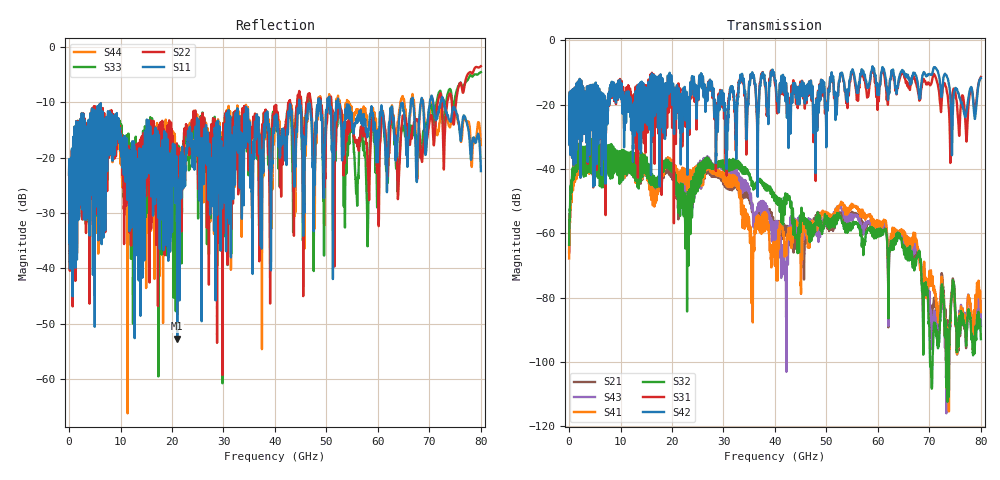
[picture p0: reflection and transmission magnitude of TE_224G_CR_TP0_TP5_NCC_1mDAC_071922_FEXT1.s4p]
!! Reference: tracy_3df_01a_2207
!! CHANNEL DESCRIPTION: TP0_TP5 CR Channel using 1meter DAC, CABLED NCC Host
!! MODEL DESCRIPTION: s4p, FEXT1
!! CONNECTOR DESCRIPTION: OSFP 200G OTB, NCC Socket
!! CABLE DESCRIPTION: 1meter 26AWG Cable
!! MODEL STATUS: Developmental
!! PORT DEFINITIONS:
!! Port  1  ----->  Side A  Side B  <-----  Port  2
!! Port  3  ----->  Side A  Side B  <-----  Port  4
# GHz S MA R 50
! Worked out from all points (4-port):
!   8000 points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, 10 MHz to 80 GHz, reference 50 ohm
!   strongest paths, dB at 10 MHz, 20.01 GHz, 40.01 GHz, 60.01 GHz, 80 GHz:
!     S42: -24.5, -18.5, -12.5, -15.2, -11.7
!     S31: -24.5, -26.1, -13.7, -17.6, -11.4
!     S32: -63.7, -39.3, -48.6, -60.8, -92.9
!     S41: -67.8, -38.5, -65.3, -58.1, -84.5
!     S43: -66.0, -38.7, -68.9, -59.4, -88.6
!     S21: -65.9, -41.3, -57.8, -59.5, -88.9
!   lowest |S11| = -52.7 dB at 21.01 GHz (marker M1), VSWR 1.00, Z = 50 + j0.231 ohm
!   |S11| at or under -10 dB: start of sweep to 44.68 GHz; 52.32 GHz to 66.38 GHz (14.06 GHz wide, 23.7 % of centre); 72.83 GHz to end of sweep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
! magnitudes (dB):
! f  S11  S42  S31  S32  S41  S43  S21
! 10 MHz  -23.1  -24.5  -24.5  -63.7  -67.8  -66.0  -65.9
! 1.96 GHz  -15.3  -18.0  -18.0  -32.1  -36.1  -33.8  -33.8
! 21.01 GHz  -52.7  -15.8  -17.3  -44.5  -40.1  -41.9  -44.6
! 35.71 GHz  -25.2  -11.4  -11.4  -44.8  -78.1  -52.5  -53.2
! 41.89 GHz  -17.7  -12.4  -13.2  -54.1  -67.3  -71.5  -60.7
! 55.26 GHz  -15.6  -10.0  -10.7  -56.6  -51.3  -54.6  -53.7
! 80 GHz  -22.4  -11.7  -11.4  -92.9  -84.5  -88.6  -88.9
